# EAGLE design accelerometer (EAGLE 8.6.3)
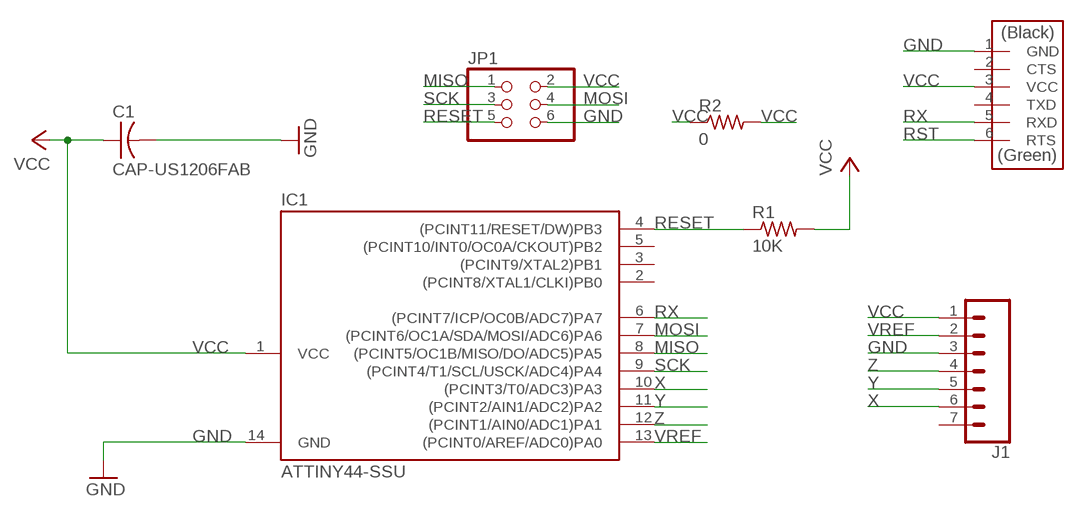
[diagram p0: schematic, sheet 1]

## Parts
C1  CAP-US1206FAB  [C1206FAB]
IC1  ATTINY44-SSU  [SOIC14]
J1  CONN_07LONGPADS  [1X07_LONGPADS]
JP1  PINHD-2X3-SMD  [2X03SMD]
R1  10K  RES-US1206FAB  [R1206FAB]
R2  0  RES-US1206FAB  [R1206FAB]
U$1  FTDI-SMD-HEADER  [1X06SMD]

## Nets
GND: C1.2 IC1.14(GND) J1.3 JP1.6 U$1.1(GND)
MISO: IC1.8((PCINT5/OC1B/MISO/DO/ADC5)PA5) JP1.1
MOSI: IC1.7((PCINT6/OC1A/SDA/MOSI/ADC6)PA6) JP1.4
RESET: IC1.4((PCINT11/RESET/DW)PB3) JP1.5 R1.1
RST: U$1.6(RTS)
RX: IC1.6((PCINT7/ICP/OC0B/ADC7)PA7) U$1.5(RXD)
SCK: IC1.9((PCINT4/T1/SCL/USCK/ADC4)PA4) JP1.3
VCC: C1.1 IC1.1(VCC) J1.1 JP1.2 R1.2 R2.1 R2.2 U$1.3(VCC)
VREF: IC1.13((PCINT0/AREF/ADC0)PA0) J1.2
X: IC1.10((PCINT3/T0/ADC3)PA3) J1.6
Y: IC1.11((PCINT2/AIN1/ADC2)PA2) J1.5
Z: IC1.12((PCINT1/AIN0/ADC1)PA1) J1.4
Unconnected: IC1.2((PCINT8/XTAL1/CLKI)PB0) IC1.3((PCINT9/XTAL2)PB1) IC1.5((PCINT10/INT0/OC0A/CKOUT)PB2) J1.7 U$1.2(CTS) U$1.4(TXD)

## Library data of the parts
C1 = fab:CAP-US
IC1 = fab:ATTINY44
J1 = SparkFun-Connectors:CONN_07: Multi connection point. Often used as Generic Header-pin footprint for 0.1 inch spaced/style header connections On any of the 0.1 inch spaced packages, you can populate with these: Break Away Headers - Straight (PRT-00116) Break Away Male Headers - Right Angle (PRT-00553) Female Headers (PRT-00115)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
JP1 = fab:PINHD-2X3-SMD: PIN HEADER
R1 R2 = fab:RES-US: Resistor (US Symbol)
U$1 = fab:FTDI-SMD-HEADER

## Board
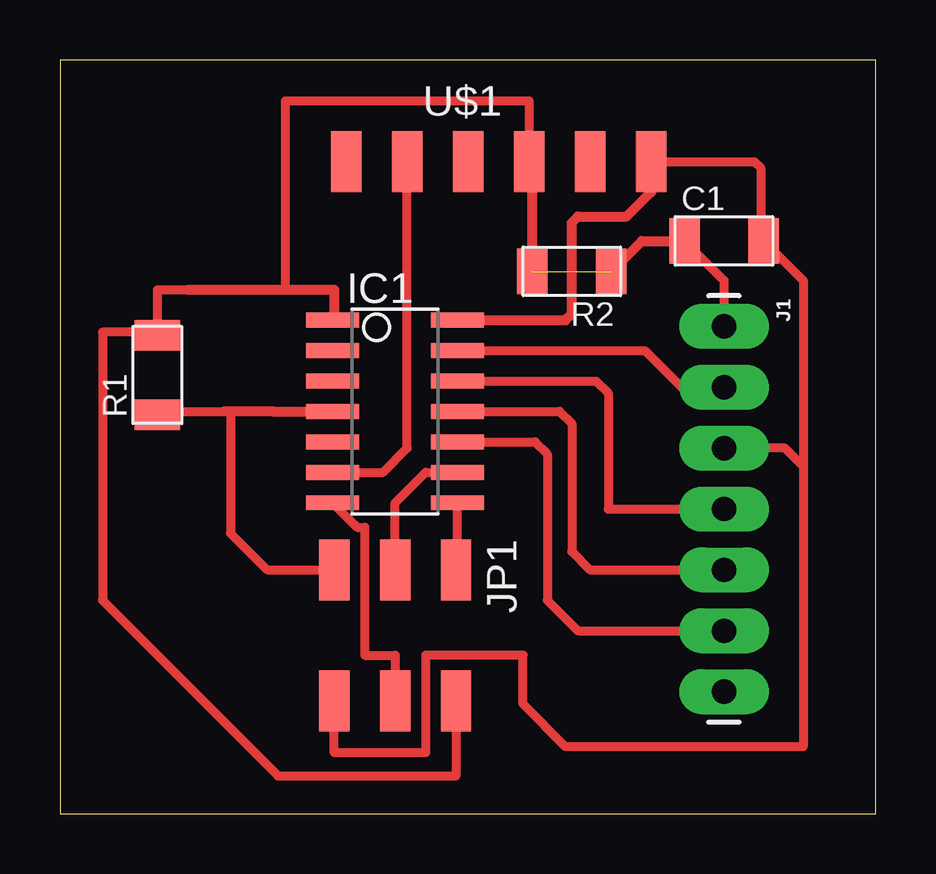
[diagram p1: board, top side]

Size 34.02 x 31.42 mm. Coordinates in mm from the lower left corner, seen from the top.
Outline: 0,0 34.02,0 34.02,31.42 0,31.42 0,0
Copper layers (1*16): Top 0.035mm / dielectric 1.5mm / Bottom 0.035mm
Design rules "default *": minimum track width 15mil, minimum drill 0.79mm, track to track 0.41mm, track to pad 0.4mm, pad to pad 0.4mm, via to via 0.4mm, smd to smd 0.4mm, copper to edge 40mil, drill to drill 6mil, minimum pad ring 10mil, minimum via ring 8mil, stop-mask expansion 4mil, vias tented up to drill 0mil, thermal gap 10mil

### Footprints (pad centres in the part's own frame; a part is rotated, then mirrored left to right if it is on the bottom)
C1206FAB = smd 1.27 x 1.905: 1 -1.651,0; 2 1.651,0
SOIC14 = smd 0.61 x 2.21: 1 -3.81,-2.603; 2 -2.54,-2.603; 3 -1.27,-2.603; 4 0,-2.603; 5 1.27,-2.603; 6 2.54,-2.603; 7 3.81,-2.603; 8 3.81,2.603; 9 2.54,2.603; 10 1.27,2.603; 11 0,2.603; 12 -1.27,2.603; 13 -2.54,2.603; 14 -3.81,2.603
1X07_LONGPADS = drill 1.016 pad 1.88 long: 1 0,0; 2 2.54,0; 3 5.08,0; 4 7.62,0; 5 10.16,0; 6 12.7,0; 7 15.24,0
2X03SMD = smd 2.54 x 1.27: 1 -2.54,2.54; 2 2.92,2.54; 3 -2.54,0; 4 2.92,0; 5 -2.54,-2.54; 6 2.92,-2.54
R1206FAB = smd 1.27 x 1.905: 1 -1.651,0; 2 1.651,0
1X06SMD = smd 2.54 x 1.27: 1 0,6.35; 2 0,3.81; 3 0,1.27; 4 0,-1.27; 5 0,-3.81; 6 0,-6.35

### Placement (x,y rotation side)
C1  27.69,23.88 0 top
IC1  13.97,16.76 270 top
J1  27.69,20.32 270 top
JP1  13.97,7.62 270 top
R1  4.06,18.29 90 top
R2  21.34,22.61 180 top
U$1  18.29,27.18 270 top

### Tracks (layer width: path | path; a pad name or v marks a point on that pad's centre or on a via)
GND
  Top 0.381: 30.99,14.48 30.99,2.79 21.08,2.79 19.3,4.57 19.3,6.6 15.24,6.6 15.24,2.54 11.43,2.54 JP1.6 | 30.99,14.48 30.23,15.24 J1.3 | 30.99,14.48 30.99,22.23 C1.2 29.21,24 29.21,26.92 28.96,27.18 U$1.1
  Top 0.406: IC1.14 21.08,20.57 21.34,20.83 21.34,24.64 21.59,24.89 23.62,24.89 24.64,25.91 U$1.1
MISO
  Top 0.381: JP1.1 16.57,10.22 IC1.8
MOSI
  Top 0.381: IC1.7 12.3,12.02 12.31,12.02 12.39,11.94 12.7,11.94 12.7,6.6 13.97,6.6 JP1.4
RESET
  Top 0.381: R1.1 4.06,16.76 7.11,16.76 7.11,11.68 8.64,10.16 JP1.5
  Top 0.406: 6.86,16.76 7.11,16.76 8.89,16.76 IC1.4
RX
  Top 0.381: IC1.6 13.46,14.22 14.48,15.24 U$1.5
SCK
  Top 0.381: JP1.3 13.97,12.95 15.24,14.22 IC1.9
VCC  (1 unrouted)
  Top 0.381: 5.59,21.84 4.06,21.84 R1.2 4.06,20.07 1.78,20.07 1.78,8.89 9.09,1.57 16.51,1.57 JP1.2 | 9.4,21.84 9.4,29.72 19.56,29.72 U$1.3 | C1.1 27.69,22.23 J1.1
  Top 0.406: IC1.1 11.43,20.57 11.43,21.84 9.4,21.84 5.59,21.84 5.33,21.84 | R2.1 24.26,23.88 C1.1 | U$1.3 19.68,27.05 R2.2
VREF
  Top 0.381: IC1.13 24.38,19.3 25.91,17.78 J1.2
X
  Top 0.381: IC1.10 19.81,15.49 20.32,14.99 20.32,8.89 21.59,7.62 J1.6
Y
  Top 0.381: IC1.11 20.83,16.76 21.34,16.26 21.34,10.92 22.1,10.16 J1.5
Z
  Top 0.381: J1.4 22.86,12.7 22.86,17.53 22.35,18.03 IC1.12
